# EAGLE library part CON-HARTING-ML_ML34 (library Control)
HARTING
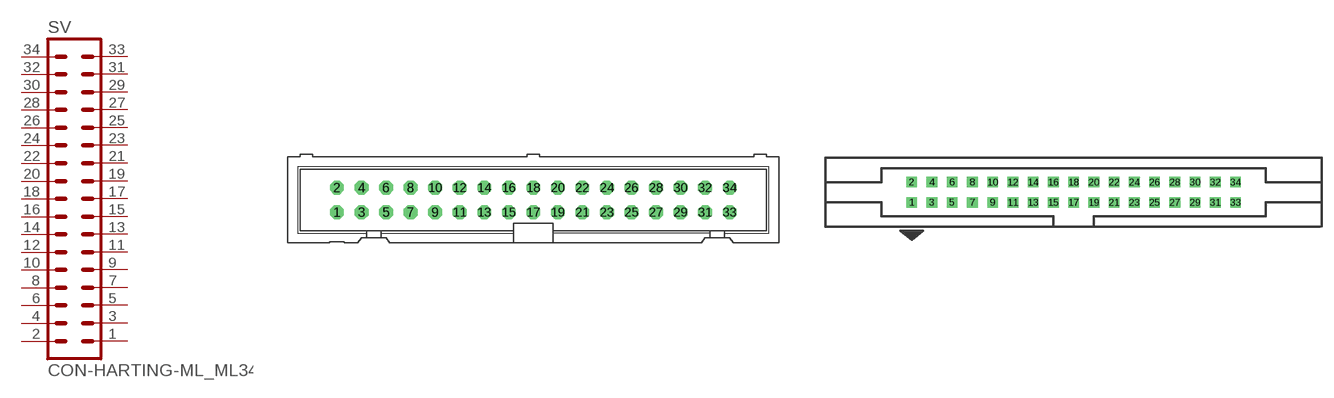
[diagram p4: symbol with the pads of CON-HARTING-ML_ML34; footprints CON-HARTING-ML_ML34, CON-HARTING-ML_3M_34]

Designator prefix SV

## CON-HARTING-ML_ML34 (OC_FARNELL: unknown; OC_NEWARK: unknown)  [CON-HARTING-ML_ML34]
1  1  pas
2  2  pas
3  3  pas
4  4  pas
5  5  pas
6  6  pas
7  7  pas
8  8  pas
9  9  pas
10  10  pas
11  11  pas
12  12  pas
13  13  pas
14  14  pas
15  15  pas
16  16  pas
17  17  pas
18  18  pas
19  19  pas
20  20  pas
21  21  pas
22  22  pas
23  23  pas
24  24  pas
25  25  pas
26  26  pas
27  27  pas
28  28  pas
29  29  pas
30  30  pas
31  31  pas
32  32  pas
33  33  pas
34  34  pas

## CON-HARTING-ML_ML343M (OC_FARNELL: unknown; OC_NEWARK: unknown)  [CON-HARTING-ML_3M_34]
Pads as for CON-HARTING-ML_ML34

## CON-HARTING-ML_ML343ML (OC_FARNELL: unknown; OC_NEWARK: unknown)  [CON-HARTING-ML_3M_34L]
Pads as for CON-HARTING-ML_ML34

## CON-HARTING-ML_ML34L (OC_FARNELL: unknown; OC_NEWARK: unknown)  [CON-HARTING-ML_ML34L]
Pads as for CON-HARTING-ML_ML34

## Footprint CON-HARTING-ML_ML34 (pad centres in mm)
HARTING
drill 0.914 octagon: 1 -20.32,-1.27; 2 -20.32,1.27; 3 -17.78,-1.27; 4 -17.78,1.27; 5 -15.24,-1.27; 6 -15.24,1.27; 7 -12.7,-1.27; 8 -12.7,1.27; 9 -10.16,-1.27; 10 -10.16,1.27; 11 -7.62,-1.27; 12 -7.62,1.27; 13 -5.08,-1.27; 14 -5.08,1.27; 15 -2.54,-1.27; 16 -2.54,1.27; 17 0,-1.27; 18 0,1.27; 19 2.54,-1.27; 20 2.54,1.27; 21 5.08,-1.27; 22 5.08,1.27; 23 7.62,-1.27; 24 7.62,1.27; 25 10.16,-1.27; 26 10.16,1.27; 27 12.7,-1.27; 28 12.7,1.27; 29 15.24,-1.27; 30 15.24,1.27; 31 17.78,-1.27; 32 17.78,1.27; 33 20.32,-1.27; 34 20.32,1.27

## Footprint CON-HARTING-ML_3M_34 (pad centres in mm)
3M
drill 0.813 square: 1 -20.32,-1.27; 2 -20.32,1.27; 3 -17.78,-1.27; 4 -17.78,1.27; 5 -15.24,-1.27; 6 -15.24,1.27; 7 -12.7,-1.27; 8 -12.7,1.27; 9 -10.16,-1.27; 10 -10.16,1.27; 11 -7.62,-1.27; 12 -7.62,1.27; 13 -5.08,-1.27; 14 -5.08,1.27; 15 -2.54,-1.27; 16 -2.54,1.27; 17 0,-1.27; 18 0,1.27; 19 2.54,-1.27; 20 2.54,1.27; 21 5.08,-1.27; 22 5.08,1.27; 23 7.62,-1.27; 24 7.62,1.27; 25 10.16,-1.27; 26 10.16,1.27; 27 12.7,-1.27; 28 12.7,1.27; 29 15.24,-1.27; 30 15.24,1.27; 31 17.78,-1.27; 32 17.78,1.27; 33 20.32,-1.27; 34 20.32,1.27

## Footprint CON-HARTING-ML_3M_34L (pad centres in mm)
3M
drill 0.813 square: 1 -20.32,-5.08; 2 -20.32,-2.54; 3 -17.78,-5.08; 4 -17.78,-2.54; 5 -15.24,-5.08; 6 -15.24,-2.54; 7 -12.7,-5.08; 8 -12.7,-2.54; 9 -10.16,-5.08; 10 -10.16,-2.54; 11 -7.62,-5.08; 12 -7.62,-2.54; 13 -5.08,-5.08; 14 -5.08,-2.54; 15 -2.54,-5.08; 16 -2.54,-2.54; 17 0,-5.08; 18 0,-2.54; 19 2.54,-5.08; 20 2.54,-2.54; 21 5.08,-5.08; 22 5.08,-2.54; 23 7.62,-5.08; 24 7.62,-2.54; 25 10.16,-5.08; 26 10.16,-2.54; 27 12.7,-5.08; 28 12.7,-2.54; 29 15.24,-5.08; 30 15.24,-2.54; 31 17.78,-5.08; 32 17.78,-2.54; 33 20.32,-5.08; 34 20.32,-2.54
hole 2.54 at -26.238,-3.277
hole 2.54 at 26.238,-3.277

## Footprint CON-HARTING-ML_ML34L (pad centres in mm)
HARTING
drill 0.914 octagon: 1 -20.32,-1.27; 2 -20.32,1.27; 3 -17.78,-1.27; 4 -17.78,1.27; 5 -15.24,-1.27; 6 -15.24,1.27; 7 -12.7,-1.27; 8 -12.7,1.27; 9 -10.16,-1.27; 10 -10.16,1.27; 11 -7.62,-1.27; 12 -7.62,1.27; 13 -5.08,-1.27; 14 -5.08,1.27; 15 -2.54,-1.27; 16 -2.54,1.27; 17 0,-1.27; 18 0,1.27; 19 2.54,-1.27; 20 2.54,1.27; 21 5.08,-1.27; 22 5.08,1.27; 23 7.62,-1.27; 24 7.62,1.27; 25 10.16,-1.27; 26 10.16,1.27; 27 12.7,-1.27; 28 12.7,1.27; 29 15.24,-1.27; 30 15.24,1.27; 31 17.78,-1.27; 32 17.78,1.27; 33 20.32,-1.27; 34 20.32,1.27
